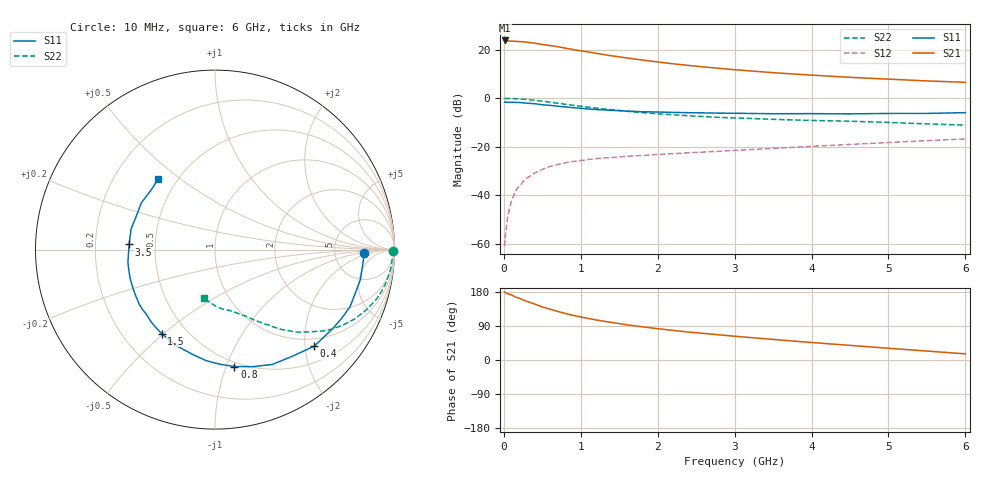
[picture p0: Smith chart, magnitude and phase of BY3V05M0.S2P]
! SIEMENS Small Signal Semiconductors
! BFY420
! Si NPN RF SIEGET Grounded Emitter Transistor in MICRO-X
! VCE = 3 V  IC = 5 mA
! Common Emitter S-Parameters:  October  1996
# GHz  S  MA  R  50
!  f  S11  S21  S12  S22
! GHz  MAG  ANG  MAG  ANG  MAG  ANG  MAG  ANG
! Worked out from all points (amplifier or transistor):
!   36 points, 10 MHz to 6 GHz, reference 50 ohm
!   highest |S21| = 23.8 dB at 10 MHz (marker M1)
!   |S21| within 3 dB of that: start of sweep to 772.2 MHz
!   unconditionally stable (mu >= 1): 3.166 GHz to end of sweep
!   at 250 MHz: K = 0.12, MSG = 28.8 dB, |S12| = -34.4 dB
!   at 1.4 GHz: K = 0.52, MSG = 20.9 dB, |S12| = -24.5 dB
!   at 6 GHz: K = 1.13, MAG = 9.4 dB, |S12| = -16.8 dB
!   S11 on the Smith chart (normalised r, x): 10 MHz: 11, -1; 400 MHz: 0.83, -2.20; 800 MHz: 0.46, -1.07; 1.5 GHz: 0.36, -0.49; 3.5 GHz: 0.35, +0.03; 6 GHz: 0.40, +0.42
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0.01  0.8325 -1.4  15.46 179.8  0.0009 85.6  0.9913 -0.5
0.02  0.8299 -2.7  15.45 177.6  0.0015 83.6  0.9829 -1.0
0.05  0.8275 -5.9  15.09 174.9  0.0037 85.4  0.9885 -2.9
0.1  0.8271 -11.6  15.01 171.6  0.0078 84.4  0.9857 -5.9
0.15  0.8186 -17.3  14.84 166.4  0.0121 80.1  0.977 -8.7
0.3  0.7907 -33.6  14.24 154.7  0.0228 72.4  0.9427 -16.9
0.4  0.7717 -44.2  13.61 147.8  0.0288 66.8  0.906 -21.9
0.5  0.7339 -54.1  12.79 140.0  0.0343 62.7  0.869 -26.4
0.6  0.7151 -63.5  12.17 134.2  0.0393 58.9  0.8291 -30.4
0.7  0.6852 -72.2  11.49 128.2  0.0433 55.7  0.7906 -34.0
0.8  0.6602 -80.6  10.74 122.7  0.0469 51.8  0.7507 -37.2
0.9  0.6391 -87.6  10.06 117.8  0.0499 49.8  0.7151 -39.7
1.1  0.5997 -101.1  8.965 109.6  0.055 45.9  0.6538 -44.7
1.3  0.5758 -112.7  7.923 102.4  0.0591 43.0  0.6019 -48.3
1.5  0.5544 -122.5  7.115 96.2  0.0619 41.1  0.558 -51.6
1.8  0.5263 -136.3  6.1 87.6  0.0664 39.0  0.5055 -55.5
2.2  0.5104 -150.5  5.114 78.1  0.0721 37.4  0.4566 -60.2
2.8  0.493 -167.2  4.119 66.4  0.081 36.2  0.4028 -65.9
3.5  0.4794 176.6  3.354 54.3  0.0927 34.7  0.3674 -72.1
4.5  0.4767 156.8  2.692 38.6  0.1119 31.2  0.3362 -81.9
5.5  0.4863 137.5  2.27 23.6  0.1338 26.1  0.2964 -95.1
6  0.5046 128.8  2.125 16.2  0.145 22.9  0.2792 -103.2
